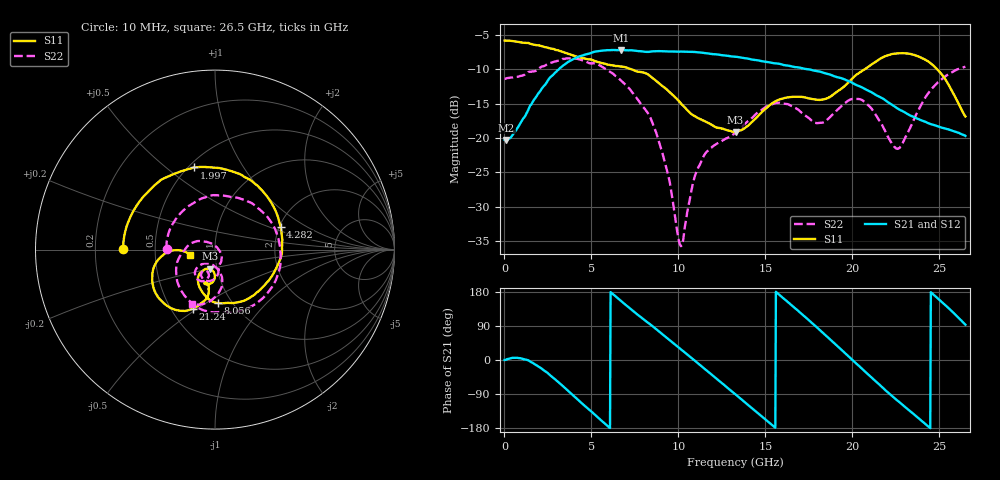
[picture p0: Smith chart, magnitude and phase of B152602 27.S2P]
!  2-Port S-parameters saved by WinCal
! VAR MeasName=S-Parameters (CALIBRATED_DATA) read from VNA (N5242A)
! VAR MeasDate=2016-1-5 16:29:33
! VAR NAME=B152602 27
! VAR FILENAME=B152602 27.S2P
! VAR DATE=2016-1-5 16:29:33
! VAR PHYS_PORTS=1,2
# Hz S DB R 50
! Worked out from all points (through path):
!   801 points, 10 MHz to 26.5 GHz, reference 50 ohm
!   highest |S21| = -7.18 dB at 6.699 GHz (marker M1); lowest = -20.3 dB at 109.3 MHz (marker M2)
!   lowest |S11| = -19.1 dB at 13.29 GHz (marker M3), VSWR 1.25, Z = 46.3 - j10 ohm
!   |S11| at or under -10 dB: 7.294 GHz to 20.71 GHz (13.41 GHz wide, 95.8 % of centre); 24.87 GHz to end of sweep
!   |S22| runs from -35.7 to -8.4 dB; largest |S21 - S12| = 0.003
!   S11 on the Smith chart (normalised r, x): 10 MHz: 0.32, +0.00; 1.997 GHz: 0.53, +0.63; 4.282 GHz: 2.03, +0.61; 8.056 GHz: 0.86, -0.56; 21.24 GHz: 0.64, -0.48; 26.5 GHz: 0.75, -0.04
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1e7  -5.83 179.5  -20.25 0.1  -20.24 -0.1  -11.39 179.6
1.093375e8  -5.81 175.8  -20.28 0.9  -20.27 0.9  -11.31 173.9
1.99675e9  -6.50 104.5  -13.41 -18.4  -13.40 -18.4  -9.85 59.8
3.155688e9  -7.32 60.1  -9.91 -60.5  -9.91 -60.4  -8.70 -5.8
4.281512e9  -8.24 19.3  -8.16 -107.2  -8.17 -107.1  -8.53 -60.6
4.447075e9  -8.37 13.7  -8.03 -114.1  -8.02 -114.0  -8.67 -67.6
5.639125e9  -9.12 -24.8  -7.29 -162.5  -7.28 -162.4  -9.69 -111.5
6.698725e9  -9.61 -53.5  -7.18 156.0  -7.19 156.0  -11.65 -144.9
8.056338e9  -10.52 -87.1  -7.46 105.2  -7.44 105.4  -15.72 177.9
8.851038e9  -11.98 -105.3  -7.36 76.6  -7.33 76.5  -20.22 150.8
1.014242e10  -14.97 -121.6  -7.43 28.8  -7.40 28.7  -35.71 41.1
1.14007e10  -17.42 -119.4  -7.60 -19.2  -7.57 -19.4  -22.90 -60.5
1.3255e10  -19.11 -104.8  -8.18 -89.6  -8.17 -89.8  -19.24 -79.8
1.328811e10  -19.14 -104.3  -8.19 -90.8  -8.19 -91.0  -19.16 -79.7
1.547354e10  -14.82 -94.1  -9.12 -175.0  -9.07 -175.0  -15.01 -100.0
1.769208e10  -14.31 -107.8  -10.12 97.0  -10.09 97.1  -17.52 -118.0
1.951326e10  -12.55 -98.5  -11.43 21.1  -11.41 21.1  -15.04 -106.2
2.123511e10  -9.08 -110.6  -13.55 -51.9  -13.51 -52.0  -16.19 -133.8
2.209604e10  -7.92 -123.6  -14.88 -87.4  -14.80 -87.8  -20.07 -128.7
2.275829e10  -7.67 -135.0  -15.93 -113.3  -15.89 -113.8  -21.27 -98.0
2.451325e10  -9.15 -165.1  -17.97 178.9  -17.96 178.4  -13.02 -81.9
2.65e10  -16.85 -168.9  -19.68 93.2  -19.67 93.1  -9.63 -112.9
